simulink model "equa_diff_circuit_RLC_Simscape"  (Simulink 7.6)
settings: Solver=ode15s  StartTime=0.0  StopTime=0.14  RelTol=1e-3
InitFcn:
  | R=1;
  | L=0.01;
  | C=1e-3;
StopFcn:
  | close all
  | load x1_et_x2.mat
  | plot(x(1,:),x(2,:),x(1,:),x(3,:))
  | %axis([0 3 0 1200])
  | grid
  | title('x1 (tension aux bornes de C) et x2 (courant dans la bobine L)')
  | xlabel('temps')
libraries: fl_lib x7, nesl_utility x4

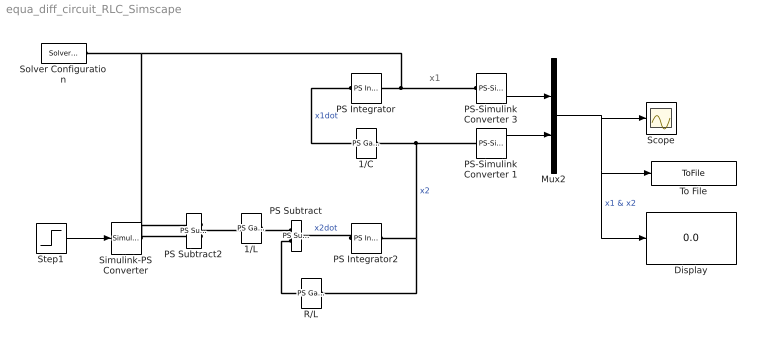
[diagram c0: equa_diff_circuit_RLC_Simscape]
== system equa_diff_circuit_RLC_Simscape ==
  note: x1
  1/C : fl_lib/Physical Signals/Functions/PS Gain  DialogController=NetworkEngine.DynNeDlgSource  SystemSampleTime=-1  gain=1/C  LocalVarLogging=[]
  1/L : fl_lib/Physical Signals/Functions/PS Gain  DialogController=NetworkEngine.DynNeDlgSource  SystemSampleTime=-1  gain=1/L  LocalVarLogging=[]
  Display : Display
  Mux2 : Mux  Inputs=2
  PS Integrator : fl_lib/Physical Signals/Linear Operators/PS Integrator  DialogController=NetworkEngine.DynNeDlgSource  SystemSampleTime=-1  x0=0  x_Log=off  LocalVarNames=|x  LocalVarDescs=|x  LocalVarLogging=0
  PS Integrator2 : fl_lib/Physical Signals/Linear Operators/PS Integrator  DialogController=NetworkEngine.DynNeDlgSource  SystemSampleTime=-1  x0=0  x_Log=off  LocalVarNames=|x  LocalVarDescs=|x  LocalVarLogging=0
  PS Subtract : fl_lib/Physical Signals/Functions/PS Subtract  DialogController=NetworkEngine.DynNeDlgSource  SystemSampleTime=-1  LocalVarLogging=[]
  PS Subtract2 : fl_lib/Physical Signals/Functions/PS Subtract  DialogController=NetworkEngine.DynNeDlgSource  SystemSampleTime=-1  LocalVarLogging=[]
  PS-Simulink Converter 1 : nesl_utility/PS-Simulink Converter  DialogController=NetworkEngine.DynNeUtilDlgSource  SystemSampleTime=-1  PhysicalDomain=network_engine_domain  LeftPortType=input  RightPortType=output  SubClassName=ps_output  Unit=1  AffineConversion=off
  PS-Simulink Converter 3 : nesl_utility/PS-Simulink Converter  DialogController=NetworkEngine.DynNeUtilDlgSource  SystemSampleTime=-1  PhysicalDomain=network_engine_domain  LeftPortType=input  RightPortType=output  SubClassName=ps_output  Unit=1  AffineConversion=off
  R/L : fl_lib/Physical Signals/Functions/PS Gain  DialogController=NetworkEngine.DynNeDlgSource  SystemSampleTime=-1  gain=R/L  LocalVarLogging=[]
  Scope : Scope
  Simulink-PS Converter : nesl_utility/Simulink-PS Converter  DialogController=NetworkEngine.DynNeUtilDlgSource  SystemSampleTime=-1  PhysicalDomain=network_engine_domain  LeftPortType=input  RightPortType=output  SubClassName=ps_input  Unit=1  AffineConversion=off  InputFilterTimeConstant=.001  UdotUserProvided=0
  Solver Configuration : nesl_utility/Solver Configuration  DialogController=NetworkEngine.DynNeUtilDlgSource  SystemSampleTime=-1  PhysicalDomain=network_engine_domain  LeftPortType=input  RightPortType=generic  SubClassName=solver  Accelerate=off  Profile=off  ResidualTolerance=1e-9  MaxNonlinIter=12  MaxModeIter=2  DoFixedCost=off  UseLocalSampling=off  DoDC=off  LinearAlgebra=Sparse  LocalSolverSampleTime=.001  LocalSolverChoice=NE_BACKWARD_EULER_ADVANCER  UseLocalSolver=off
  Step1 : Step  Time=0.02  SampleTime=0
  To File : ToFile  Filename=x1_et_x2  MatrixName=x
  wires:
  PS-Simulink Converter 3/1 -> Mux2/1
  PS-Simulink Converter 1/1 -> Mux2/2
  Mux2/1 -> Scope/1, To File/1, Display/1  "x1 & x2"
  Step1/1 -> Simulink-PS Converter/1
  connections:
  1/C/RConn1 -- PS Integrator/LConn1  "x1dot"
  Solver Configuration/RConn1 -- PS Integrator/RConn1 -- PS-Simulink Converter 3/LConn1 -- PS Subtract2/LConn2
  R/L/RConn1 -- PS Subtract/LConn2
  PS Integrator2/LConn1 -- PS Subtract/RConn1  "x2dot"
  Simulink-PS Converter/RConn1 -- PS Subtract2/LConn1
  1/L/RConn1 -- PS Subtract/LConn1
  1/L/LConn1 -- PS Subtract2/RConn1
  PS Integrator2/RConn1 -- PS-Simulink Converter 1/LConn1 -- 1/C/LConn1 -- R/L/LConn1  "x2"
